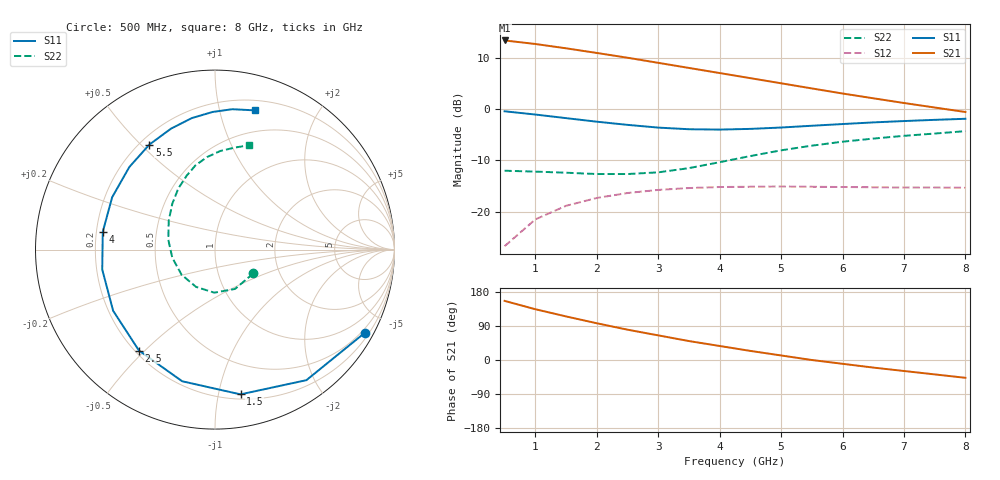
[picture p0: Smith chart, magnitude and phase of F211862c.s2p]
!ATF-21186
!S-PARAMETERS at Vds=2V  Id=20mA.  LAST UPDATED 01-30-98
# ghz s ma r 50
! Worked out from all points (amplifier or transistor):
!   16 points, 500 MHz to 8 GHz, reference 50 ohm
!   highest |S21| = 13.4 dB at 500 MHz (marker M1)
!   |S21| within 3 dB of that: start of sweep to 2.3 GHz
!   unconditionally stable (mu >= 1): 5.755 GHz to end of sweep
!   at 1.5 GHz: K = 0.40, MSG = 15.4 dB, |S12| = -18.9 dB
!   at 4.5 GHz: K = 0.91, MSG = 10.6 dB, |S12| = -15.1 dB
!   at 8 GHz: K = 1.05, MAG = 6.0 dB, |S12| = -15.3 dB
!   lowest NFmin = 0.33 dB at 500 MHz
!   S11 on the Smith chart (normalised r, x): 500 MHz: 0.36, -3.83; 1.5 GHz: 0.24, -1.16; 2.5 GHz: 0.22, -0.48; 4 GHz: 0.23, +0.07; 5.5 GHz: 0.24, +0.53; 8 GHz: 0.29, +1.29
0.5  0.955 -29.0  4.698 156.0  0.046 71.0  0.251 -32.0
1  0.888 -55.0  4.34 134.0  0.084 57.0  0.246 -63.0
1.5  0.819 -80.0  3.938 115.0  0.114 44.0  0.24 -91.0
2  0.756 -104.0  3.547 97.0  0.136 33.0  0.233 -117.0
2.5  0.704 -127.0  3.186 80.0  0.152 23.0  0.233 -143.0
3  0.662 -149.0  2.84 65.0  0.163 14.0  0.242 -169.0
3.5  0.638 -170.0  2.532 50.0  0.17 6.0  0.266 168.0
4  0.633 171.0  2.257 37.0  0.174 -1.0  0.304 148.0
4.5  0.643 153.0  2.012 24.0  0.175 -7.0  0.349 133.0
5  0.663 136.0  1.793 12.0  0.176 -13.0  0.397 121.0
5.5  0.69 122.0  1.597 0.0  0.175 -19.0  0.441 111.0
6  0.717 110.0  1.425 -10.0  0.174 -24.0  0.482 103.0
6.5  0.744 100.0  1.28 -20.0  0.173 -28.0  0.517 95.0
7  0.767 91.0  1.151 -29.0  0.172 -33.0  0.55 87.0
7.5  0.788 83.0  1.04 -38.0  0.172 -37.0  0.579 79.0
8  0.807 74.0  0.94 -47.0  0.171 -41.0  0.611 72.0
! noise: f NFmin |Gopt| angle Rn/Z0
0.5  0.33  0.95  13  1.543
1  0.37  0.88  28  0.659
2  0.45  0.77  64  0.294
3  0.52  0.65  103  0.124
3.5  0.56  0.62  123  0.079
4.5  0.63  0.59  168  0.024
5.5  0.7  0.64  -150  0.044
6  0.74  0.68  -134  0.089
7  0.81  0.77  -107  0.289
8  0.89  0.83  -84  0.654
